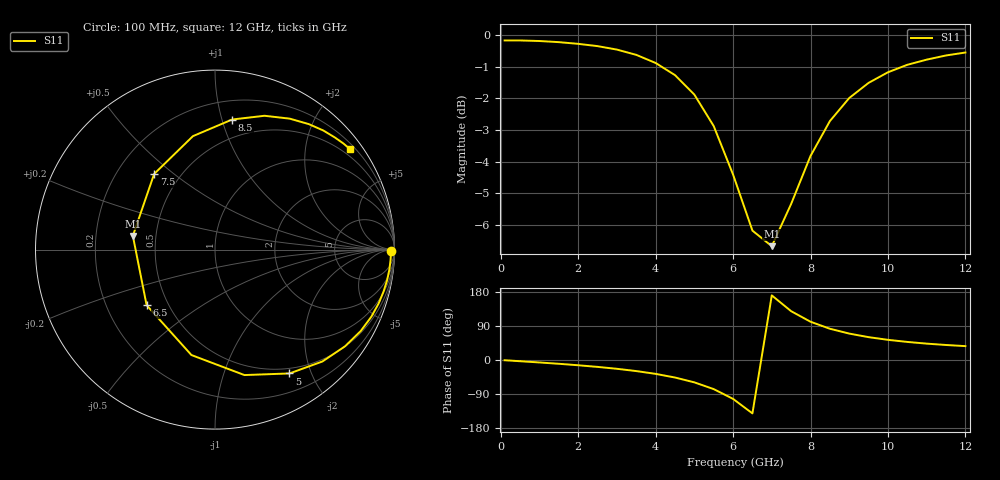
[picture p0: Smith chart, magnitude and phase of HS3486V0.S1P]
!HSCH-3486 zero bias Schottky diode
!S-parameters at zero bias.  Last updated 6/7/94
# ghz s ma r 50
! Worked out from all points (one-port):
!   25 points, 100 MHz to 12 GHz, reference 50 ohm
!   lowest |S11| = -6.7 dB at 7 GHz (marker M1), VSWR 2.73, Z = 18.4 + j3.59 ohm
!   |S11| at or under -10 dB: nowhere
!   S11 on the Smith chart (normalised r, x): 100 MHz: 78, -40; 5 GHz: 0.43, -1.69; 6.5 GHz: 0.38, -0.31; 7.5 GHz: 0.36, +0.43; 8.5 GHz: 0.35, +1.08; 12 GHz: 0.32, +2.99
0.1  0.98 -0.6
0.5  0.98 -3.2
1  0.978 -6.5
1.5  0.974 -10.0
2  0.968 -13.9
2.5  0.96 -18.2
3  0.948 -23.2
3.5  0.93 -29.2
4  0.903 -36.6
4.5  0.864 -46.2
5  0.805 -59.0
5.5  0.718 -76.8
6  0.602 -102.6
6.5  0.491 -140.9
7  0.464 170.5
7.5  0.541 128.8
8  0.644 101.0
8.5  0.731 82.5
9  0.795 69.7
9.5  0.84 60.3
10  0.873 53.2
10.5  0.897 47.7
11  0.914 43.2
11.5  0.928 39.6
12  0.938 36.6
